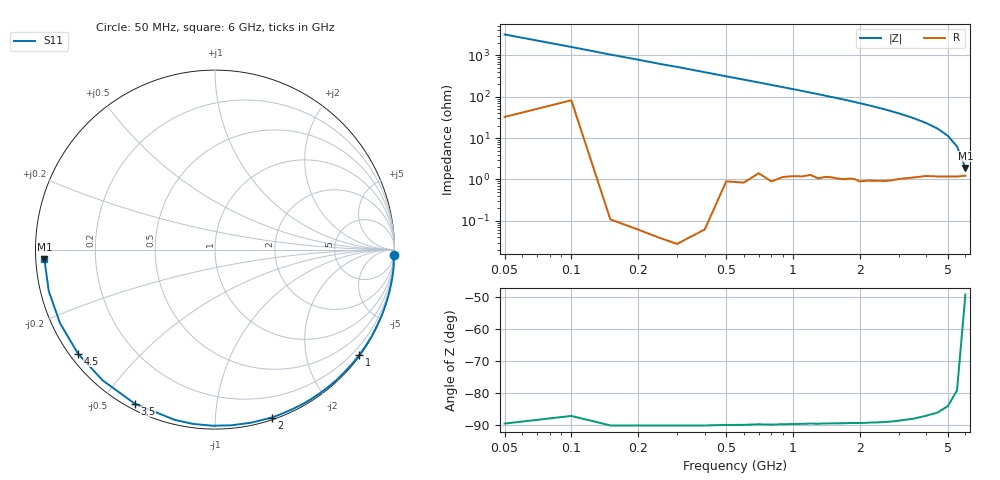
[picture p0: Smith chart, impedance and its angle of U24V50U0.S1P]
! SIEMENS Discrete & RF Semiconductors
! BBY52-02W
! Si Tuning Diode in SCD-80
! VR = 4.5 V
! S-Parameters:  September  1997
# GHz  S  MA  R  50
!  f  S11
! GHz  MAG  ANG
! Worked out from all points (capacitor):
!   34 points, 50 MHz to 6 GHz, reference 50 ohm
!   read as one part to ground: C = 1 pF near 50 MHz
!   lowest |Z| = 1.9 ohm at 6 GHz (marker M1)
!   S11 on the Smith chart (normalised r, x): 50 MHz: 1, -64; 1 GHz: 0.02, -3.05; 2 GHz: 0.02, -1.39; 3.5 GHz: 0.02, -0.61; 4.5 GHz: 0.02, -0.34; 6 GHz: 0.02, -0.03
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0.05  0.9997 -1.8
0.1  0.9968 -3.6
0.15  1 -5.5
0.2  1 -7.3
0.25  1 -9.2
0.3  1 -10.9
0.4  1 -14.6
0.6  0.9988 -21.9
0.8  0.9977 -29.2
1  0.9953 -36.3
1.1  0.9945 -39.9
1.3  0.9933 -47.0
1.4  0.9916 -50.6
1.6  0.9903 -57.6
1.7  0.9896 -60.9
1.8  0.9881 -64.5
2  0.9878 -71.3
2.2  0.9852 -78.0
2.4  0.9834 -84.5
2.6  0.9814 -90.9
2.8  0.9787 -97.2
3  0.9751 -103.2
3.5  0.9678 -117.5
4  0.9607 -130.7
4.5  0.9585 -142.8
5  0.9558 -154.6
5.5  0.9546 -166.0
6  0.9518 -176.7
